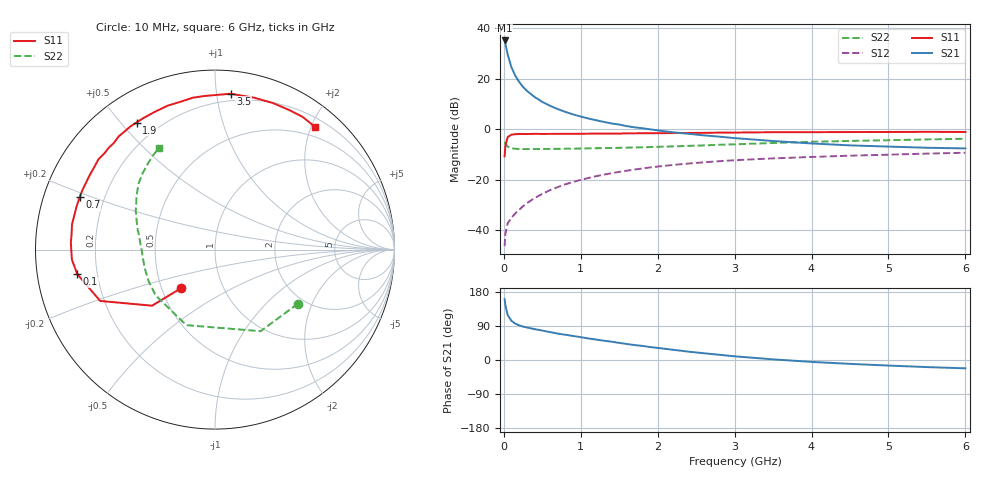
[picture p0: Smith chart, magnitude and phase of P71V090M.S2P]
! SIEMENS Small Signal Semiconductors
! BFP196
! Si NPN RF Bipolar Junction Transistor in SOT143
! VCE = 1 V  IC = 90 mA
! Common Emitter S-Parameters:  May  1996
# GHz  S  MA  R  50
!  f  S11  S21  S12  S22
! GHz  MAG  ANG  MAG  ANG  MAG  ANG  MAG  ANG
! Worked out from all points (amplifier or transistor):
!   36 points, 10 MHz to 6 GHz, reference 50 ohm
!   highest |S21| = 35.2 dB at 10 MHz (marker M1)
!   |S21| within 3 dB of that: start of sweep to 32 MHz
!   unconditionally stable (mu >= 1): start of sweep to 12.67 MHz; 196.4 MHz to end of sweep
!   at 250 MHz: K = 1.06, MAG = 22.1 dB, |S12| = -30.5 dB
!   at 1.4 GHz: K = 1.18, MAG = 7.3 dB, |S12| = -17.5 dB
!   at 6 GHz: K = 1.07, MAG = -0.7 dB, |S12| = -9.3 dB
!   S11 on the Smith chart (normalised r, x): 10 MHz: 0.62, -0.30; 100 MHz: 0.12, -0.09; 700 MHz: 0.11, +0.18; 1.9 GHz: 0.12, +0.55; 3.5 GHz: 0.15, +1.09; 6 GHz: 0.33, +2.05
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0.01  0.2891 -131.5  57.46 160.7  0.0048 64.3  0.5515 -33.1
0.02  0.4697 -138.3  49.52 144.6  0.0084 57.6  0.5209 -60.8
0.05  0.7008 -155.9  30.28 118.7  0.0137 45.4  0.4503 -110.8
0.1  0.7793 -169.9  16.7 103.0  0.0177 47.8  0.4178 -142.4
0.15  0.799 -175.9  11.4 95.9  0.0215 52.3  0.4095 -154.8
0.2  0.8009 -179.9  8.615 91.4  0.0252 57.2  0.4053 -161.5
0.25  0.8043 176.9  6.873 88.2  0.0298 60.1  0.4046 -166.0
0.3  0.8033 174.6  5.752 85.8  0.0341 62.5  0.4037 -168.6
0.4  0.809 169.9  4.344 81.4  0.0432 64.6  0.4045 -172.7
0.5  0.8068 166.5  3.485 77.7  0.0521 65.5  0.4051 -175.5
0.6  0.8079 162.7  2.913 73.7  0.0619 65.6  0.4066 -177.5
0.7  0.8085 158.9  2.509 69.7  0.071 65.4  0.408 -179.2
0.9  0.8096 152.4  1.966 63.4  0.0902 63.3  0.4114 177.8
1.1  0.8146 145.7  1.629 56.8  0.1082 60.6  0.417 175.4
1.4  0.8199 136.1  1.301 48.4  0.1341 56.2  0.4246 172.0
1.9  0.832 121.7  0.995 34.2  0.1746 48.0  0.443 166.1
2.2  0.8375 113.6  0.868 27.0  0.1957 43.0  0.4557 162.3
2.8  0.8552 98.3  0.712 13.8  0.2321 33.4  0.491 154.1
3.5  0.8728 84.3  0.583 1.7  0.2639 22.8  0.5328 145.0
4.5  0.8781 68.5  0.478 -10.2  0.2984 10.4  0.5859 133.5
5.5  0.8861 56.5  0.429 -18.7  0.3282 -0.5  0.6272 123.7
6  0.8818 51.0  0.416 -22.0  0.3413 -6.3  0.6465 118.8
